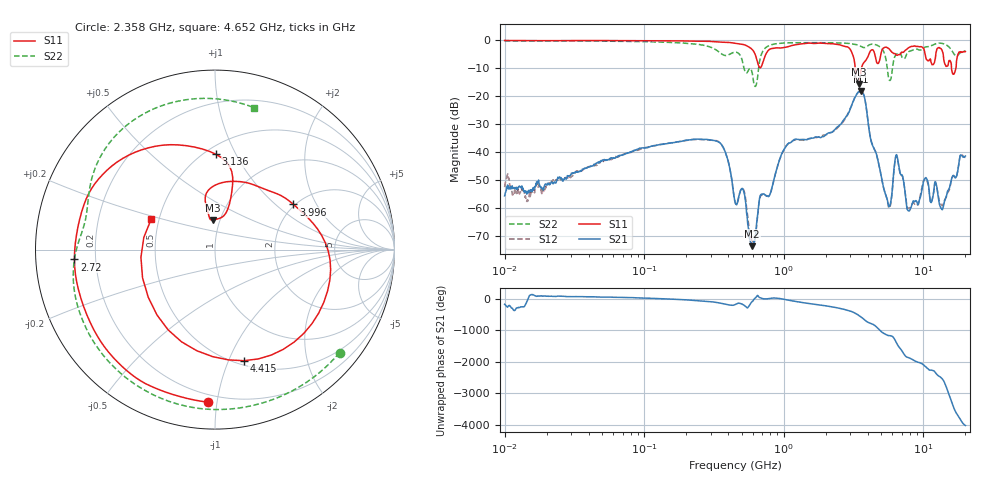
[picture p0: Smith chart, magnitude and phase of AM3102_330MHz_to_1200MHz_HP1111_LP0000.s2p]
! Date/Time: Tue, Sep 11, 2018 5:24 PM
! Network Analyzer: Agilent Technologies E8362B Rev: A.07.50.63
! Sweep from 0.010 to 20.000 GHz, 1601 Points, Sweep Type: LOG
! Power Supply: 4.949 V, 0.001 A
# Hz S DB R 50
!freq MagS11 AngS11 MagS21 AngS21 MagS12 AngS12 MagS22 AngS22
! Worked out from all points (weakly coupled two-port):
!   1601 points, 10 MHz to 20 GHz, reference 50 ohm
!   highest |S21| = -18.18 dB at 3.549 GHz (marker M1); lowest = -73.7 dB at 591.9 MHz (marker M2)
!   lowest |S11| = -15.6 dB at 3.432 GHz (marker M3), VSWR 1.40, Z = 46.1 + j15.7 ohm
!   |S11| at or under -10 dB: 3.25 GHz to 3.598 GHz (348.6 MHz wide, 10.2 % of centre); 15.91 GHz to 17.11 GHz (1.199 GHz wide, 7.26 % of centre)
!   |S22| runs from -16.5 to -0.2 dB; largest |S21 - S12| = 0.0049
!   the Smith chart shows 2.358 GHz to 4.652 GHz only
!   S11 on the Smith chart (normalised r, x): 2.358 GHz: 0.15, -0.94; 2.72 GHz: 0.12, -0.03; 3.136 GHz: 0.57, +0.84; 3.996 GHz: 1.96, +1.32; 4.415 GHz: 0.54, -1.14; 4.652 GHz: 0.45, +0.18
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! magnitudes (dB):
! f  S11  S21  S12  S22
! 10 MHz  0.0  -55.7  -52.6  -0.2
! 35.55 MHz  -0.1  -46.7  -46.8  -0.2
! 126.4 MHz  -0.2  -37.5  -37.4  -0.6
! 344.4 MHz  -0.6  -36.6  -36.5  -4.2
! 447.2 MHz  -1.0  -57.8  -57.9  -4.2
! 591.9 MHz  -3.2  -73.7  -72.2  -11.3
! 1.003 GHz  -2.6  -39.2  -39.2  -0.9
! 1.59 GHz  -1.0  -35.0  -35.0  -0.8
! 2.358 GHz  -1.4  -31.5  -31.9  -0.9
! 2.72 GHz  -2.1  -28.1  -28.5  -1.0
! 3.136 GHz  -5.5  -22.0  -22.0  -1.3
! 3.432 GHz  -15.6  -18.4  -18.5  -1.8
! 3.549 GHz  -11.9  -18.2  -18.1  -2.1
! 3.996 GHz  -5.9  -28.4  -28.2  -1.9
! 4.415 GHz  -3.9  -38.7  -38.5  -1.4
! 4.652 GHz  -8.1  -41.5  -41.5  -1.7
! 5.652 GHz  -2.9  -59.4  -59.9  -13.7
! 6.396 GHz  -5.2  -41.0  -41.2  -5.0
! 7.882 GHz  -2.6  -61.1  -60.1  -4.0
! 10.38 GHz  -5.9  -49.2  -49.4  -2.4
! 13.61 GHz  -3.6  -60.6  -59.2  -1.1
! 20 GHz  -4.0  -41.4  -42.0  -3.8
